(* Logix 5000 AddOnInstructionDefinition export BMC_AOI_PROC_BNI00HM; software revision 20.04; part 2 of 2 *)
(* tags used below, declared in another part *)
   BNI_EIP_508_Raw_Input_Data : SINT[392];
   Mapped_BNI_EIP_508_Data : BMC_UDT_PROC_BNI00HM_Data_4277US;
(* BMC_AOI_PROC_BNI00HM, continued *)

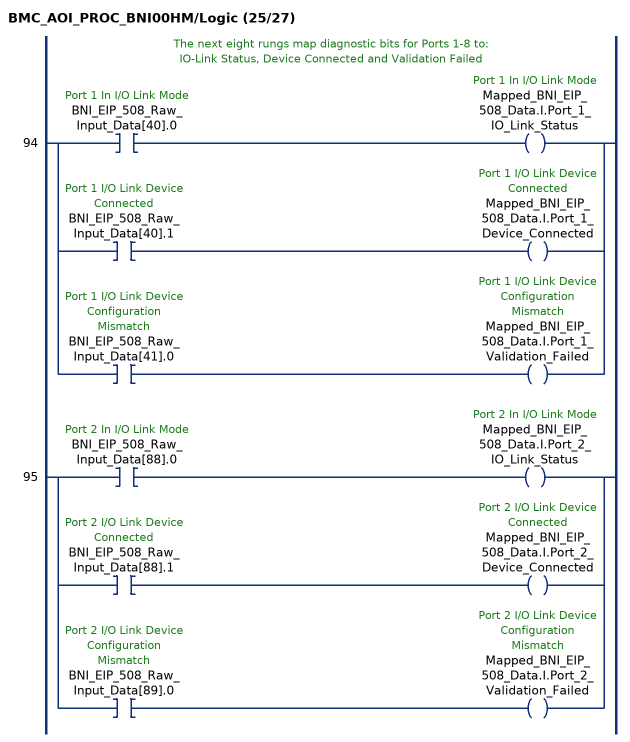
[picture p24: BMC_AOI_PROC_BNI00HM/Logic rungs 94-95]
   // The next eight rungs map diagnostic bits for Ports 1-8 to:
   // IO-Link Status, Device Connected and Validation Failed
   94: [XIC(BNI_EIP_508_Raw_Input_Data[40].0) OTE(Mapped_BNI_EIP_508_Data.I.Port_1_IO_Link_Status) ,XIC(BNI_EIP_508_Raw_Input_Data[40].1) OTE(Mapped_BNI_EIP_508_Data.I.Port_1_Device_Connected) ,XIC(BNI_EIP_508_Raw_Input_Data[41].0) OTE(Mapped_BNI_EIP_508_Data.I.Port_1_Validation_Failed) ];
   95: [XIC(BNI_EIP_508_Raw_Input_Data[88].0) OTE(Mapped_BNI_EIP_508_Data.I.Port_2_IO_Link_Status) ,XIC(BNI_EIP_508_Raw_Input_Data[88].1) OTE(Mapped_BNI_EIP_508_Data.I.Port_2_Device_Connected) ,XIC(BNI_EIP_508_Raw_Input_Data[89].0) OTE(Mapped_BNI_EIP_508_Data.I.Port_2_Validation_Failed) ];
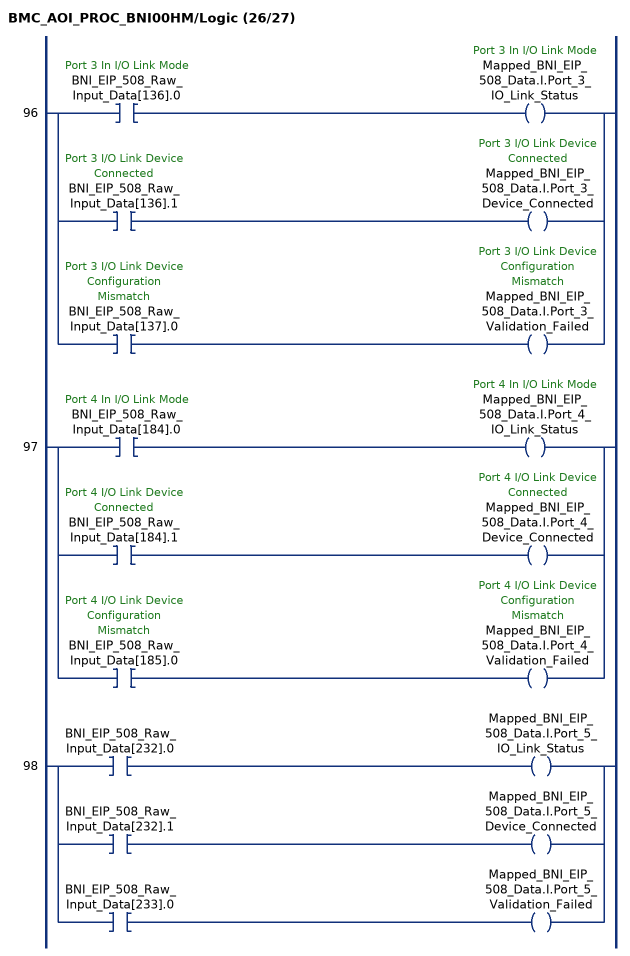
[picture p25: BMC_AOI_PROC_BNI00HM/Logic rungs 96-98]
   96: [XIC(BNI_EIP_508_Raw_Input_Data[136].0) OTE(Mapped_BNI_EIP_508_Data.I.Port_3_IO_Link_Status) ,XIC(BNI_EIP_508_Raw_Input_Data[136].1) OTE(Mapped_BNI_EIP_508_Data.I.Port_3_Device_Connected) ,XIC(BNI_EIP_508_Raw_Input_Data[137].0) OTE(Mapped_BNI_EIP_508_Data.I.Port_3_Validation_Failed) ];
   97: [XIC(BNI_EIP_508_Raw_Input_Data[184].0) OTE(Mapped_BNI_EIP_508_Data.I.Port_4_IO_Link_Status) ,XIC(BNI_EIP_508_Raw_Input_Data[184].1) OTE(Mapped_BNI_EIP_508_Data.I.Port_4_Device_Connected) ,XIC(BNI_EIP_508_Raw_Input_Data[185].0) OTE(Mapped_BNI_EIP_508_Data.I.Port_4_Validation_Failed) ];
   98: [XIC(BNI_EIP_508_Raw_Input_Data[232].0) OTE(Mapped_BNI_EIP_508_Data.I.Port_5_IO_Link_Status) ,XIC(BNI_EIP_508_Raw_Input_Data[232].1) OTE(Mapped_BNI_EIP_508_Data.I.Port_5_Device_Connected) ,XIC(BNI_EIP_508_Raw_Input_Data[233].0) OTE(Mapped_BNI_EIP_508_Data.I.Port_5_Validation_Failed) ];
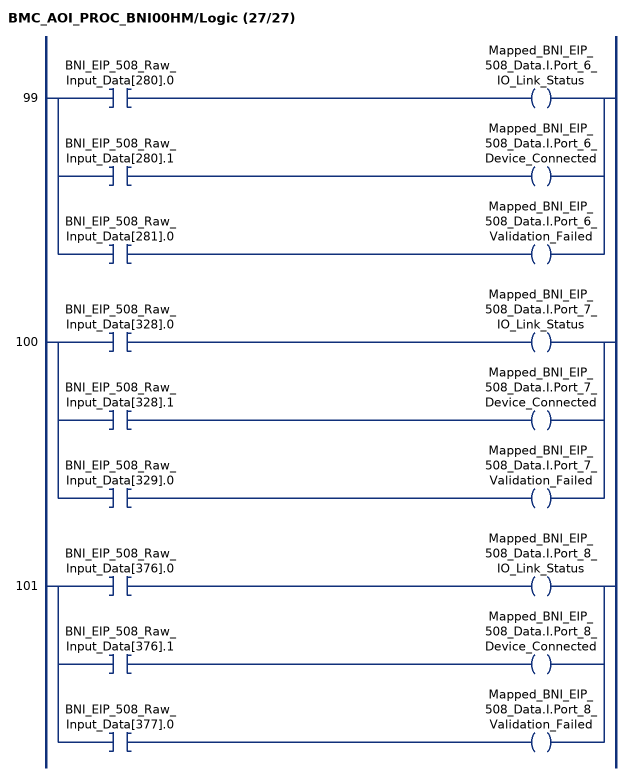
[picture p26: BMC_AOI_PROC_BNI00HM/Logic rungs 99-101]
   99: [XIC(BNI_EIP_508_Raw_Input_Data[280].0) OTE(Mapped_BNI_EIP_508_Data.I.Port_6_IO_Link_Status) ,XIC(BNI_EIP_508_Raw_Input_Data[280].1) OTE(Mapped_BNI_EIP_508_Data.I.Port_6_Device_Connected) ,XIC(BNI_EIP_508_Raw_Input_Data[281].0) OTE(Mapped_BNI_EIP_508_Data.I.Port_6_Validation_Failed) ];
   100: [XIC(BNI_EIP_508_Raw_Input_Data[328].0) OTE(Mapped_BNI_EIP_508_Data.I.Port_7_IO_Link_Status) ,XIC(BNI_EIP_508_Raw_Input_Data[328].1) OTE(Mapped_BNI_EIP_508_Data.I.Port_7_Device_Connected) ,XIC(BNI_EIP_508_Raw_Input_Data[329].0) OTE(Mapped_BNI_EIP_508_Data.I.Port_7_Validation_Failed) ];
   101: [XIC(BNI_EIP_508_Raw_Input_Data[376].0) OTE(Mapped_BNI_EIP_508_Data.I.Port_8_IO_Link_Status) ,XIC(BNI_EIP_508_Raw_Input_Data[376].1) OTE(Mapped_BNI_EIP_508_Data.I.Port_8_Device_Connected) ,XIC(BNI_EIP_508_Raw_Input_Data[377].0) OTE(Mapped_BNI_EIP_508_Data.I.Port_8_Validation_Failed) ];
END_ROUTINE
END_ADD_ON_INSTRUCTION
